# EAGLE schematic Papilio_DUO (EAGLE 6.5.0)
DATABASE: C:/Dropbox/GadgetFactory/GadgetFactory_Engineering/Libraries/GadgetFactory-PARTSDB.txt
Assembly variants: 512KB-SRAM, 1MB-SRAM, 2MB-SRAM, No-SRAM

## Sheet 1 of 4: FPGA
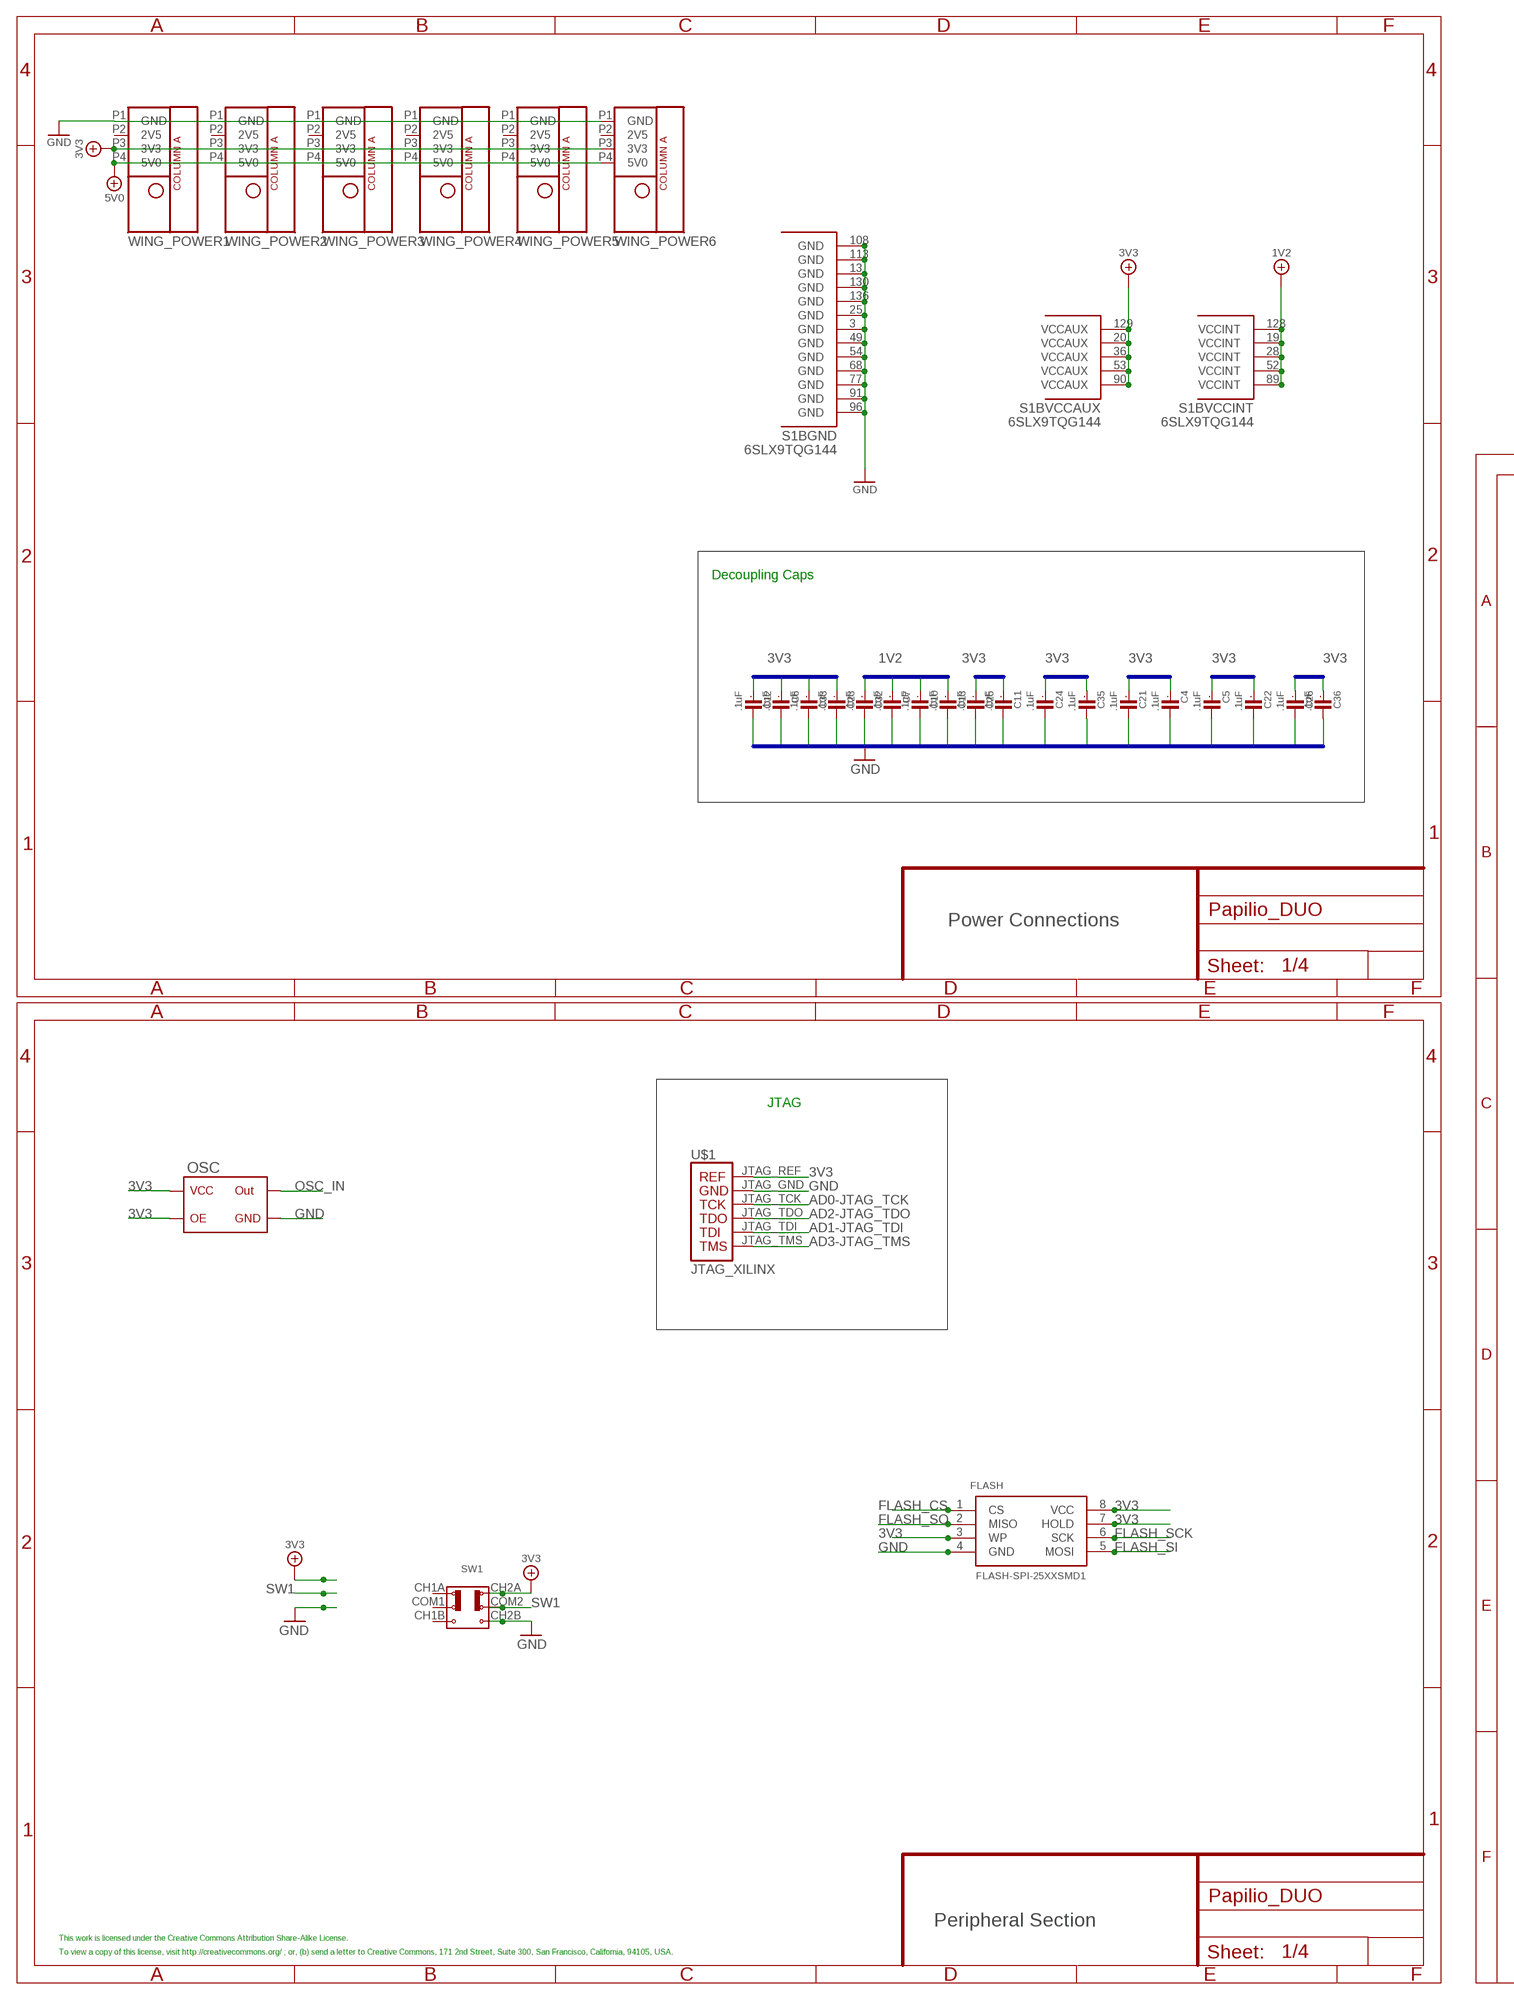
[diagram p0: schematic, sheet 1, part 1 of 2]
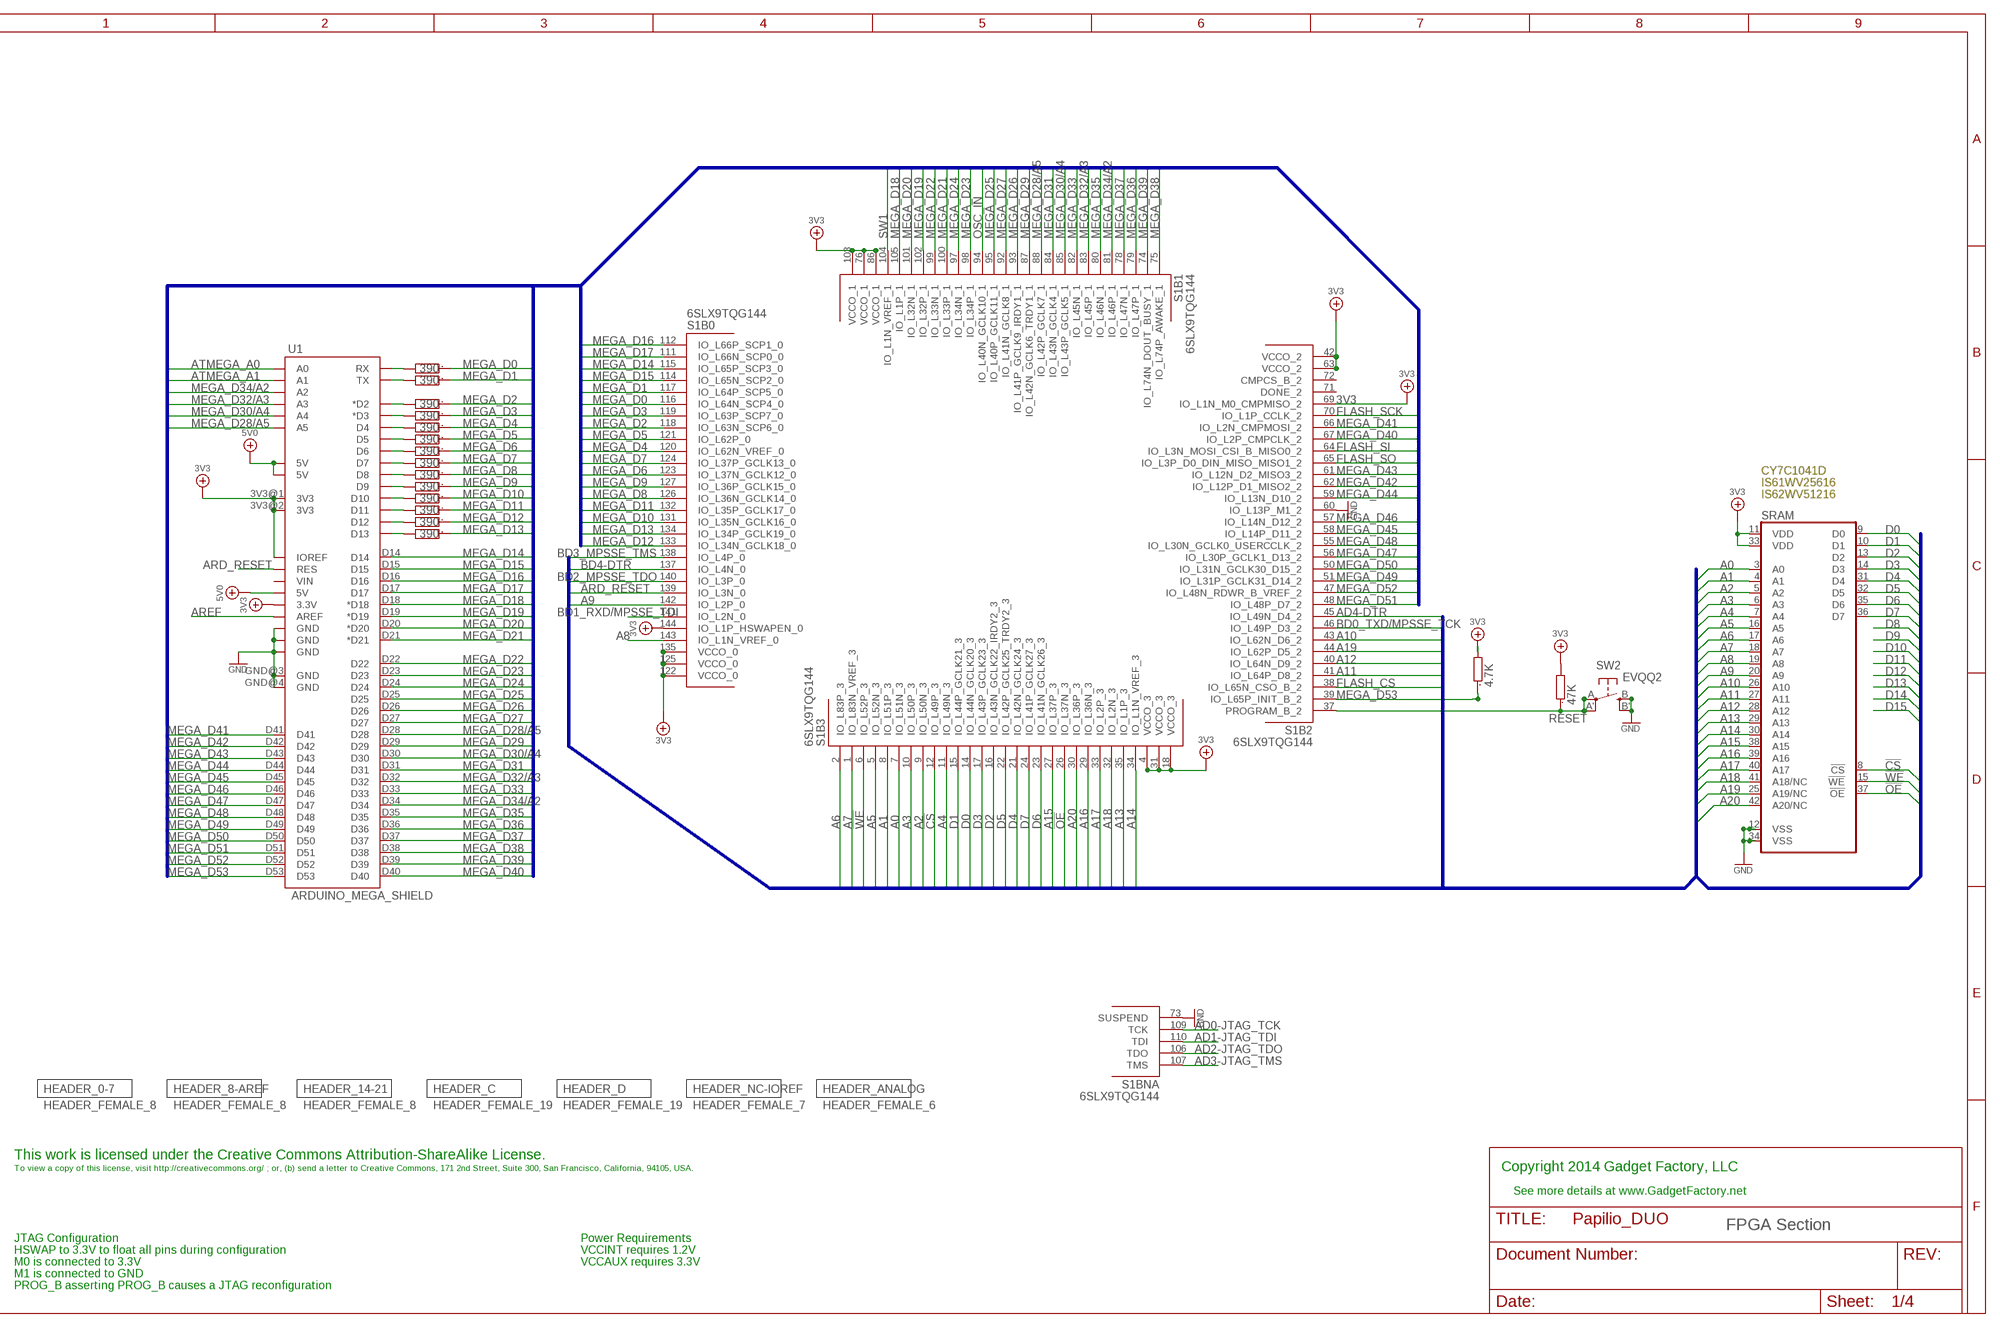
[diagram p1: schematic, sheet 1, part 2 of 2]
HEADER_0-7 (BOM-PART): BOM: INCLUDE; PARTNO: PPTC081LFBN-RC; QTY: 1
HEADER_8-AREF (BOM-PART): BOM: INCLUDE; PARTNO: PPTC081LFBN-RC; QTY: 1
HEADER_14-21 (BOM-PART): BOM: INCLUDE; PARTNO: PPTC081LFBN-RC; QTY: 1
HEADER_ANALOG (BOM-PART): BOM: INCLUDE; PARTNO: PPTC061LFBN-RC; QTY: 1
HEADER_C (BOM-PART): BOM: INCLUDE; PARTNO: PPTC191LFBN-RC; QTY: 1
HEADER_D (BOM-PART): BOM: INCLUDE; PARTNO: PPTC191LFBN-RC; QTY: 1
HEADER_NC-IOREF (BOM-PART): BOM: INCLUDE; PARTNO: PPTC071LFBN-RC; QTY: 1

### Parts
C4  .1uF  C0603  [0603]
C5  .1uF  C0603  [0603]
C6  .1uF  C0603  [0603]
C7  .1uF  C0603  [0603]
C10  .1uF  C0603  [0603]
C11  .1uF  C0603  [0603]
C12  .1uF  C0603  [0603]
C13  .1uF  C0603  [0603]
C21  .1uF  C0603  [0603]
C22  .1uF  C0603  [0603]
C23  .1uF  C0603  [0603]
C24  .1uF  C0603  [0603]
C25  .1uF  C0603  [0603]
C26  .1uF  C0603  [0603]
C32  .1uF  C0603  [0603]
C33  .1uF  C0603  [0603]
C35  .1uF  C0603  [0603]
C36  .1uF  C0603  [0603]
FLASH  FLASH-SPI-25XXSMD1  [SO08-EIAJ]
OSC  OSC1  [OSC1]
R8  390  R0603  [0603]
R9  390  R0603  [0603]
R10  390  R0603  [0603]
R11  390  R0603  [0603]
R12  390  R0603  [0603]
R13  390  R0603  [0603]
R14  390  R0603  [0603]
R15  390  R0603  [0603]
R16  390  R0603  [0603]
R17  390  R0603  [0603]
R18  390  R0603  [0603]
R19  390  R0603  [0603]
R20  390  R0603  [0603]
R21  390  R0603  [0603]
R31  47K  R0805  [0805]
R32  4.7K  R0603  [0603]
S1  6SLX9TQG144  [TQ144]
SRAM  ISSI_SRAM_8BIT  [TSOP44-II]  (variant 512KB-SRAM: 512KB-SRAM)  (variant 1MB-SRAM: 1MB-SRAM)  (variant 2MB-SRAM: 2MB-SRAM)  (not fitted in variant No-SRAM)
SW1  SWITCH-2CH-6P-3010010P1  [6P-2CH-2.54-9.1X3.5X3.2+2H]
SW2  EVQQ2  [EVQ-Q2]
U1  ARDUINO_MEGA_SHIELD  [ARDUINO_MEGA_SHIELD]
U$1  JTAG_XILINX  [JTAG]
WING_POWER1  HEADER_FEMALE_4  POWER_ONLYNOTEXT  [POWER_NO_TEXT]
WING_POWER2  HEADER_FEMALE_4  POWER_ONLYNOTEXT  [POWER_NO_TEXT]
WING_POWER3  HEADER_FEMALE_4  POWER_ONLYNOTEXT  [POWER_NO_TEXT]
WING_POWER4  HEADER_FEMALE_4  POWER_ONLYNOTEXT  [POWER_NO_TEXT]
WING_POWER5  HEADER_FEMALE_4  POWER_ONLYNOTEXT  [POWER_NO_TEXT]
WING_POWER6  HEADER_FEMALE_4  POWER_ONLYNOTEXT  [POWER_NO_TEXT]

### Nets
1V2: C7.1 C10.1 C13.1 C32.1 S1.19(BVCCINT:VCCINT) S1.28(BVCCINT:VCCINT) S1.52(BVCCINT:VCCINT) S1.89(BVCCINT:VCCINT) S1.128(BVCCINT:VCCINT) ; also sheet 2
3V3: C4.1 C5.1 C6.1 C11.1 C12.1 C21.1 C22.1 C23.1 C24.1 C25.1 C26.1 C33.1 C35.1 C36.1 FLASH.3(WP) FLASH.7(HOLD) FLASH.8(VCC) OSC.1@1(OE) OSC.4@4(VCC) R31.2 R32.2 S1.4(B3:VCCO_3) S1.18(B3:VCCO_3) S1.20(BVCCAUX:VCCAUX) S1.31(B3:VCCO_3) S1.36(BVCCAUX:VCCAUX) S1.42(B2:VCCO_2) S1.53(BVCCAUX:VCCAUX) S1.63(B2:VCCO_2) S1.69(B2:IO_L1N_M0_CMPMISO_2) S1.76(B1:VCCO_1) S1.86(B1:VCCO_1) S1.90(BVCCAUX:VCCAUX) S1.103(B1:VCCO_1) S1.122(B0:VCCO_0) S1.125(B0:VCCO_0) S1.129(BVCCAUX:VCCAUX) S1.135(B0:VCCO_0) S1.144(B0:IO_L1P_HSWAPEN_0) SRAM.11(VDD) SRAM.33(VDD) SW1.CH2A U1.3.3V U1.3V3@1(3V3) U1.3V3@2(3V3) U1.IOREF U$1.JTAG_REF WING_POWER1.P3(3V3) WING_POWER2.P3(3V3) WING_POWER3.P3(3V3) WING_POWER4.P3(3V3) WING_POWER5.P3(3V3) WING_POWER6.P3(3V3) ; also sheet 2,3,4
5V0: U1.5V@0(5V) U1.5V@1(5V) U1.5V@2(5V) WING_POWER1.P4(5V0) WING_POWER2.P4(5V0) WING_POWER3.P4(5V0) WING_POWER4.P4(5V0) WING_POWER5.P4(5V0) WING_POWER6.P4(5V0) ; also sheet 2
!CS: S1.12(B3:IO_L49P_3) SRAM.8(!CS)
!OE: S1.26(B3:IO_L37N_3) SRAM.37(!OE)
!WE: S1.6(B3:IO_L52P_3) SRAM.15(!WE)
A0: S1.7(B3:IO_L51N_3) SRAM.3(A0)
A1: S1.8(B3:IO_L51P_3) SRAM.4(A1)
A2: S1.9(B3:IO_L50N_3) SRAM.5(A2)
A3: S1.10(B3:IO_L50P_3) SRAM.6(A3)
A4: S1.11(B3:IO_L49N_3) SRAM.7(A4)
A5: S1.5(B3:IO_L52N_3) SRAM.16(A5)
A6: S1.2(B3:IO_L83P_3) SRAM.17(A6)
A7: S1.1(B3:IO_L83N_VREF_3) SRAM.18(A7)
A8: S1.143(B0:IO_L1N_VREF_0) SRAM.19(A8)
A9: S1.142(B0:IO_L2P_0) SRAM.20(A9)
A10: S1.43(B2:IO_L62N_D6_2) SRAM.26(A10)
A11: S1.41(B2:IO_L64P_D8_2) SRAM.27(A11)
A12: S1.40(B2:IO_L64N_D9_2) SRAM.28(A12)
A13: S1.35(B3:IO_L1P_3) SRAM.29(A13)
A14: S1.34(B3:IO_L1N_VREF_3) SRAM.30(A14)
A15: S1.27(B3:IO_L37P_3) SRAM.38(A15)
A16: S1.29(B3:IO_L36N_3) SRAM.39(A16)
A17: S1.33(B3:IO_L2P_3) SRAM.40(A17)
A18: S1.32(B3:IO_L2N_3) SRAM.41(A18/NC)
A19: S1.44(B2:IO_L62P_D5_2) SRAM.25(A19/NC)
A20: S1.30(B3:IO_L36P_3) SRAM.42(A20/NC)
AD0-JTAG_TCK: S1.109(BNA:TCK) U$1.JTAG_TCK ; also sheet 3
AD1-JTAG_TDI: S1.110(BNA:TDI) U$1.JTAG_TDI ; also sheet 3
AD2-JTAG_TDO: S1.106(BNA:TDO) U$1.JTAG_TDO ; also sheet 3
AD3-JTAG_TMS: S1.107(BNA:TMS) U$1.JTAG_TMS ; also sheet 3
AD4-DTR: S1.45(B2:IO_L49N_D4_2) ; also sheet 3
ARD_RESET: S1.139(B0:IO_L3N_0) U1.RES ; also sheet 4
AREF [aref]: U1.AREF ; also sheet 4
ATMEGA_A0: U1.A0 ; also sheet 4
ATMEGA_A1: U1.A1 ; also sheet 4
ATMEGA_D0/RX: R21.2 U1.RX ; also sheet 4
ATMEGA_D1/TX: R20.2 U1.TX ; also sheet 4
ATMEGA_D2: R19.2 U1.D2(*D2) ; also sheet 4
ATMEGA_D3: R18.2 U1.D3(*D3) ; also sheet 4
ATMEGA_D4: R17.2 U1.D4 ; also sheet 4
ATMEGA_D5*: R16.2 U1.D5 ; also sheet 4
ATMEGA_D6*: R15.2 U1.D6 ; also sheet 4
ATMEGA_D7: R14.2 U1.D7 ; also sheet 4
ATMEGA_IO8: R13.2 U1.D8 ; also sheet 4
ATMEGA_IO9*: R12.2 U1.D9 ; also sheet 4
ATMEGA_IO10*: R11.2 U1.D10 ; also sheet 4
ATMEGA_IO11*: R10.2 U1.D11 ; also sheet 4
ATMEGA_IO12: R9.2 U1.D12 ; also sheet 4
ATMEGA_IO13*: R8.2 U1.D13 ; also sheet 4
BD0_TXD/MPSSE_TCK: S1.46(B2:IO_L49P_D3_2) ; also sheet 3
BD1_RXD/MPSSE_TDI: S1.141(B0:IO_L2N_0) ; also sheet 3
BD2_MPSSE_TDO: S1.140(B0:IO_L3P_0) ; also sheet 3
BD3_MPSSE_TMS: S1.138(B0:IO_L4P_0) ; also sheet 3
BD4-DTR: S1.137(B0:IO_L4N_0) ; also sheet 3
D0: S1.14(B3:IO_L44N_GCLK20_3) SRAM.9(D0)
D1: S1.15(B3:IO_L44P_GCLK21_3) SRAM.10(D1)
D2: S1.16(B3:IO_L43N_GCLK22_IRDY2_3) SRAM.13(D2)
D3: S1.17(B3:IO_L43P_GCLK23_3) SRAM.14(D3)
D4: S1.21(B3:IO_L42N_GCLK24_3) SRAM.31(D4)
D5: S1.22(B3:IO_L42P_GCLK25_TRDY2_3) SRAM.32(D5)
D6: S1.23(B3:IO_L41N_GCLK26_3) SRAM.35(D6)
D7: S1.24(B3:IO_L41P_GCLK27_3) SRAM.36(D7)
FLASH_CS: FLASH.1(CS) S1.38(B2:IO_L65N_CSO_B_2)
FLASH_SCK: FLASH.6(SCK) S1.70(B2:IO_L1P_CCLK_2)
FLASH_SI: FLASH.5(MOSI) S1.64(B2:IO_L3N_MOSI_CSI_B_MISO0_2)
FLASH_SO: FLASH.2(MISO) S1.65(B2:IO_L3P_D0_DIN_MISO_MISO1_2)
GND: C4.2 C5.2 C6.2 C7.2 C10.2 C11.2 C12.2 C13.2 C21.2 C22.2 C23.2 C24.2 C25.2 C26.2 C32.2 C33.2 C35.2 C36.2 FLASH.4(GND) OSC.2@2(GND) S1.3(BGND:GND) S1.13(BGND:GND) S1.25(BGND:GND) S1.49(BGND:GND) S1.54(BGND:GND) S1.60(B2:IO_L13P_M1_2) S1.68(BGND:GND) S1.73(BNA:SUSPEND) S1.77(BGND:GND) S1.91(BGND:GND) S1.96(BGND:GND) S1.108(BGND:GND) S1.113(BGND:GND) S1.130(BGND:GND) S1.136(BGND:GND) SRAM.12(VSS) SRAM.34(VSS) SW1.CH2B SW2.B'(S1) SW2.B(S) U1.GND@0(GND) U1.GND@1(GND) U1.GND@2(GND) U1.GND@3(GND) U1.GND@4(GND) U$1.JTAG_GND WING_POWER1.P1(GND) WING_POWER2.P1(GND) WING_POWER3.P1(GND) WING_POWER4.P1(GND) WING_POWER5.P1(GND) WING_POWER6.P1(GND) ; also sheet 2,3,4
MEGA_D0: R21.1 S1.116(B0:IO_L64N_SCP4_0)
MEGA_D1: R20.1 S1.117(B0:IO_L64P_SCP5_0)
MEGA_D2: R19.1 S1.118(B0:IO_L63N_SCP6_0)
MEGA_D3: R18.1 S1.119(B0:IO_L63P_SCP7_0)
MEGA_D4: R17.1 S1.120(B0:IO_L62N_VREF_0)
MEGA_D5: R16.1 S1.121(B0:IO_L62P_0)
MEGA_D6: R15.1 S1.123(B0:IO_L37N_GCLK12_0)
MEGA_D7: R14.1 S1.124(B0:IO_L37P_GCLK13_0)
MEGA_D8: R13.1 S1.126(B0:IO_L36N_GCLK14_0)
MEGA_D9: R12.1 S1.127(B0:IO_L36P_GCLK15_0)
MEGA_D10: R11.1 S1.131(B0:IO_L35N_GCLK16_0)
MEGA_D11: R10.1 S1.132(B0:IO_L35P_GCLK17_0)
MEGA_D12: R9.1 S1.133(B0:IO_L34N_GCLK18_0)
MEGA_D13: R8.1 S1.134(B0:IO_L34P_GCLK19_0)
MEGA_D14: S1.115(B0:IO_L65P_SCP3_0) U1.D14 ; also sheet 4
MEGA_D15: S1.114(B0:IO_L65N_SCP2_0) U1.D15 ; also sheet 4
MEGA_D16: S1.112(B0:IO_L66P_SCP1_0) U1.D16 ; also sheet 4
MEGA_D17: S1.111(B0:IO_L66N_SCP0_0) U1.D17
MEGA_D18: S1.105(B1:IO_L1P_1) U1.D18(*D18)
MEGA_D19: S1.102(B1:IO_L32P_1) U1.D19(*D19)
MEGA_D20: S1.101(B1:IO_L32N_1) U1.D20(*D20)
MEGA_D21: S1.100(B1:IO_L33P_1) U1.D21(*D21)
MEGA_D22: S1.99(B1:IO_L33N_1) U1.D22
MEGA_D23: S1.98(B1:IO_L34P_1) U1.D23
MEGA_D24: S1.97(B1:IO_L34N_1) U1.D24
MEGA_D25: S1.95(B1:IO_L40P_GCLK11_1) U1.D25
MEGA_D26: S1.93(B1:IO_L41P_GCLK9_IRDY1_1) U1.D26
MEGA_D27: S1.92(B1:IO_L41N_GCLK8_1) U1.D27
MEGA_D28/A5: S1.88(B1:IO_L42P_GCLK7_1) U1.A5 U1.D28 ; also sheet 4
MEGA_D29: S1.87(B1:IO_L42N_GCLK6_TRDY1_1) U1.D29
MEGA_D30/A4: S1.85(B1:IO_L43P_GCLK5_1) U1.A4 U1.D30 ; also sheet 4
MEGA_D31: S1.84(B1:IO_L43N_GCLK4_1) U1.D31
MEGA_D32/A3: S1.83(B1:IO_L45P_1) U1.A3 U1.D32 ; also sheet 4
MEGA_D33: S1.82(B1:IO_L45N_1) U1.D33
MEGA_D34/A2: S1.81(B1:IO_L46P_1) U1.A2 U1.D34 ; also sheet 4
MEGA_D35: S1.80(B1:IO_L46N_1) U1.D35
MEGA_D36: S1.79(B1:IO_L47P_1) U1.D36
MEGA_D37: S1.78(B1:IO_L47N_1) U1.D37
MEGA_D38: S1.75(B1:IO_L74P_AWAKE_1) U1.D38
MEGA_D39: S1.74(B1:IO_L74N_DOUT_BUSY_1) U1.D39
MEGA_D40: S1.67(B2:IO_L2P_CMPCLK_2) U1.D40
MEGA_D41: S1.66(B2:IO_L2N_CMPMOSI_2) U1.D41
MEGA_D42: S1.62(B2:IO_L12P_D1_MISO2_2) U1.D42
MEGA_D43: S1.61(B2:IO_L12N_D2_MISO3_2) U1.D43
MEGA_D44: S1.59(B2:IO_L13N_D10_2) U1.D44
MEGA_D45: S1.58(B2:IO_L14P_D11_2) U1.D45
MEGA_D46: S1.57(B2:IO_L14N_D12_2) U1.D46
MEGA_D47: S1.56(B2:IO_L30P_GCLK1_D13_2) U1.D47
MEGA_D48: S1.55(B2:IO_L30N_GCLK0_USERCCLK_2) U1.D48
MEGA_D49: S1.51(B2:IO_L31P_GCLK31_D14_2) U1.D49
MEGA_D50: S1.50(B2:IO_L31N_GCLK30_D15_2) U1.D50
MEGA_D51: S1.48(B2:IO_L48P_D7_2) U1.D51
MEGA_D52: S1.47(B2:IO_L48N_RDWR_B_VREF_2) U1.D52
MEGA_D53: R32.1 S1.39(B2:IO_L65P_INIT_B_2) U1.D53
OSC_IN: OSC.3@3(OUT) S1.94(B1:IO_L40N_GCLK10_1)
RESET: R31.1 S1.37(B2:PROGRAM_B_2) SW2.A'(P1) SW2.A(P)
SW1: S1.104(B1:IO_L1N_VREF_1) SW1.COM2
Unconnected: S1.71(B2:DONE_2) S1.72(B2:CMPCS_B_2) SW1.CH1A SW1.CH1B SW1.COM1 U1.VIN WING_POWER1.P2(2V5) WING_POWER2.P2(2V5) WING_POWER3.P2(2V5) WING_POWER4.P2(2V5) WING_POWER5.P2(2V5) WING_POWER6.P2(2V5)

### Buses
GND
1V2
MEGA_A[0..15],MEGA_D[0..53],W1_B[1..16],OSC_IN,FLASH_SCK,FLASH_SI,FLASH_SO,FLASH_CS,USB_TXD,USB_RXD,LED1,LED2,LED3,LED4
3V3
A[0..20],D[0..15],CS,WE,OE,BE,LED4

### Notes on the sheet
- Decoupling Caps
- Power Connections
- CY7C1041D
- IS61WV25616
- IS62WV51216
- JTAG
- RESET
- This work is licensed under the Creative Commons Attribution-ShareAlike License.
- To view a copy of this license, visit http://creativecommons.org/ ; or, (b) send a letter to Creative Commons, 171 2nd Street, Suite 300, San Francisco, California, 94105, USA. | Copyright 2014 Gadget Factory, LLC
- See more details at www.GadgetFactory.net
- FPGA Section
- JTAG Configuration | Power Requirements
- HSWAP to 3.3V to float all pins during configuration | VCCINT requires 1.2V
- Peripheral Section | M0 is connected to 3.3V | VCCAUX requires 3.3V
- This work is licensed under the Creative Commons Attribution Share-Alike License. | M1 is connected to GND
- To view a copy of this license, visit http://creativecommons.org/ ; or, (b) send a letter to Creative Commons, 171 2nd Street, Suite 300, San Francisco, California, 94105, USA. | PROG_B asserting PROG_B causes a JTAG reconfiguration

## Sheet 2 of 4: Power
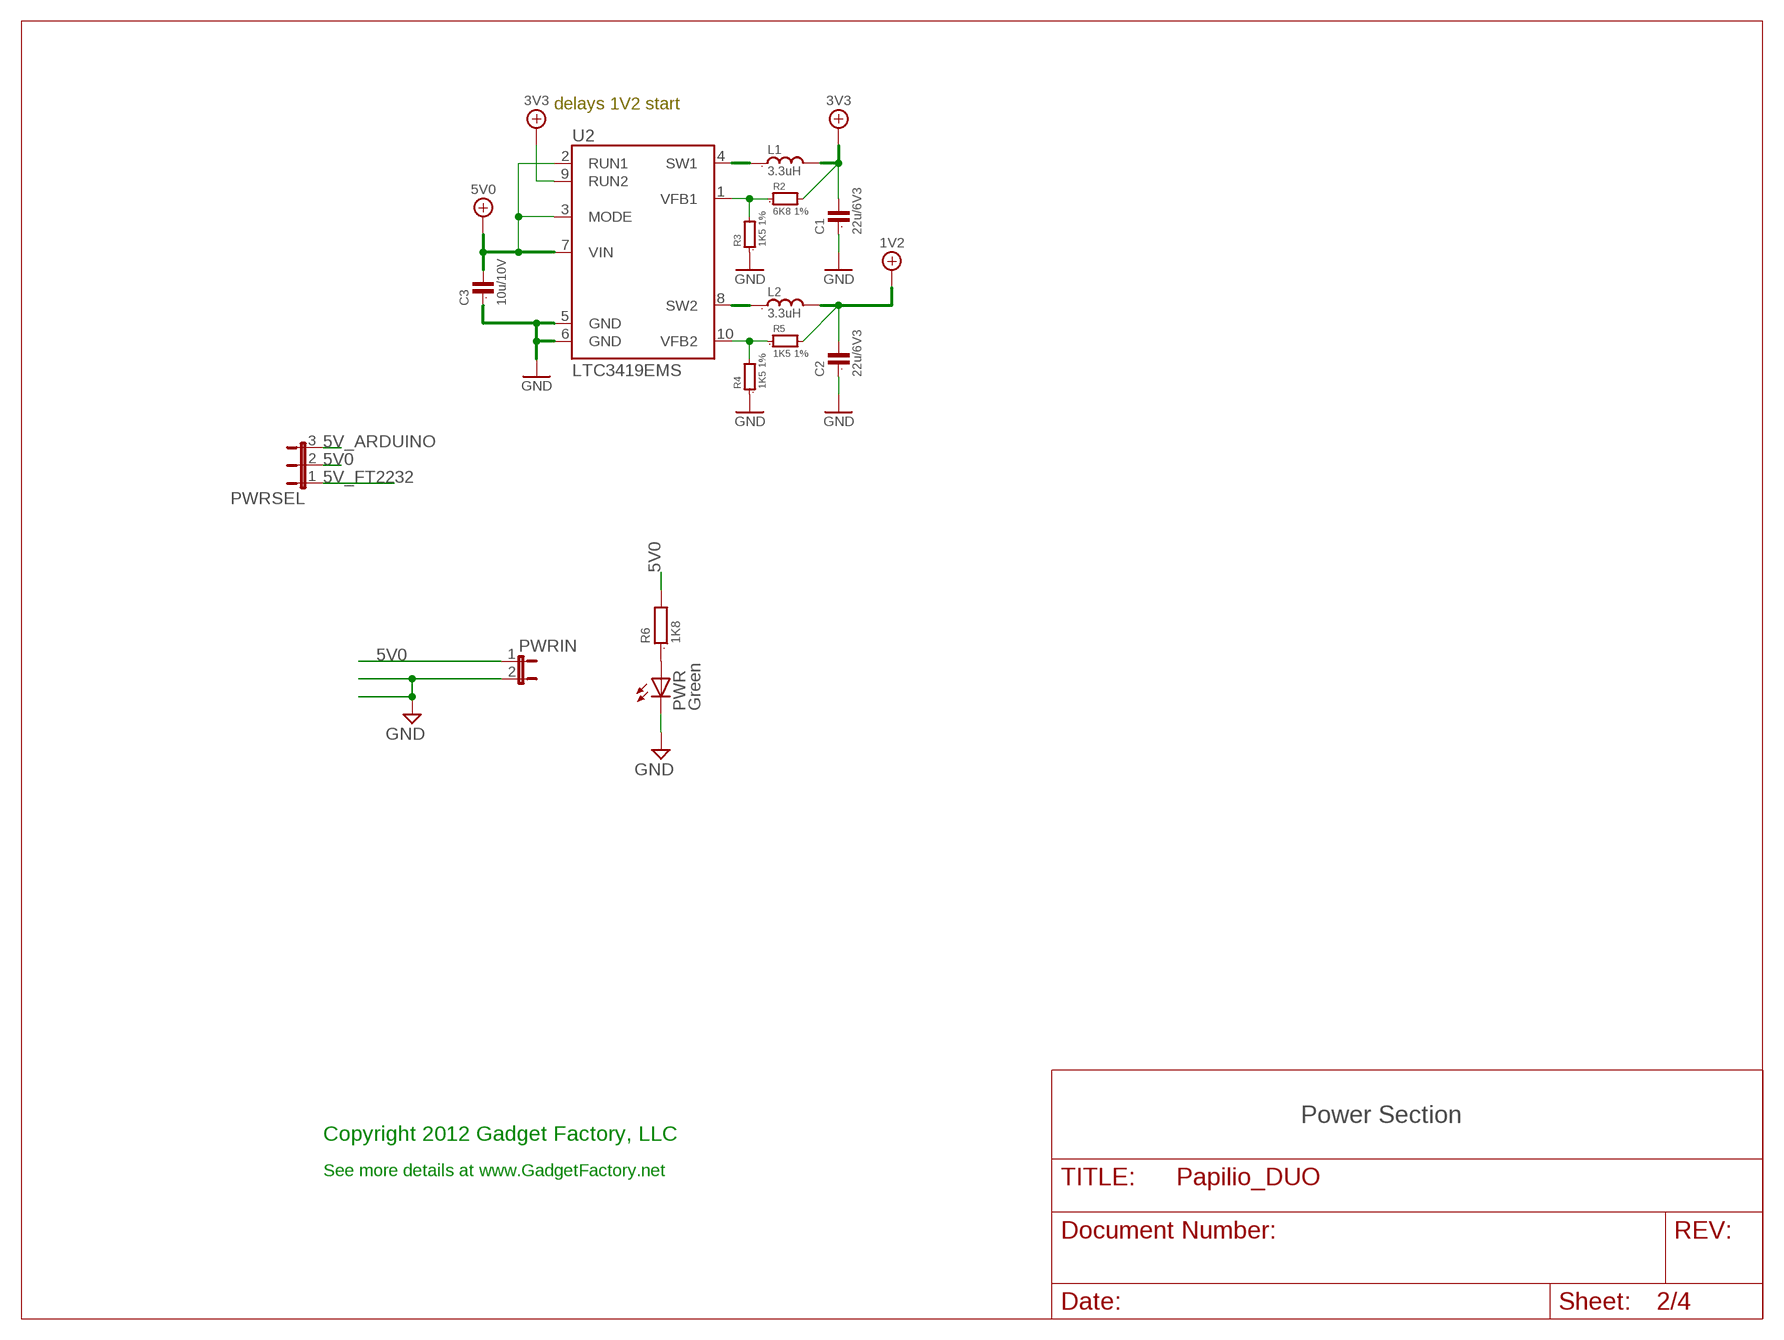
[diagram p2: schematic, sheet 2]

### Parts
C1  22u/6V3  C0805  [0805]
C2  22u/6V3  C0805  [0805]
C3  10u/10V  C0805  [0805]
L1  3.3uH  L_VLS3015  [VLS3015]
L2  3.3uH  L_VLS3015  [VLS3015]
PWR  Green  LEDCHIP-LED0805  [CHIP-LED0805]
PWRIN  JP1E  [JP1]
PWRSEL  JP2E  [JP2]
R2  6K8 1%  R-SMALL0603  [0603]
R3  1K5 1%  R-SMALL0603  [0603]
R4  1K5 1%  R-SMALL0603  [0603]
R5  1K5 1%  R-SMALL0603  [0603]
R6  1K8  R0603  [0603]
U2  LTC3419EMS  [MSOP10]

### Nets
1V2: C2.2 L2.2 R5.2 ; also sheet 1
3V3: C1.2 L1.2 R2.2 U2.9(RUN2) ; also sheet 1,3,4
5V0: C3.2 PWRIN.1 PWRSEL.2 R6.2 U2.2(RUN1) U2.3(MODE) U2.7(VIN) ; also sheet 1
5V_ARDUINO: PWRSEL.3 ; also sheet 4
5V_FT2232: PWRSEL.1 ; also sheet 3
FB_1V2: R4.2 R5.1 U2.10(VFB2)
FB_3V3: R2.1 R3.2 U2.1(VFB1)
GND: C1.1 C2.1 C3.1 PWR.C PWRIN.2 R3.1 R4.1 U2.5(GND) U2.6(GND) ; also sheet 1,3,4
N$8: PWR.A R6.1
SW_1V2: L2.1 U2.8(SW2)
SW_3V3: L1.1 U2.4(SW1)

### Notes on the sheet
- delays 1V2 start
- Power Section
- Copyright 2012 Gadget Factory, LLC
- See more details at www.GadgetFactory.net

## Sheet 3 of 4: FT2232H
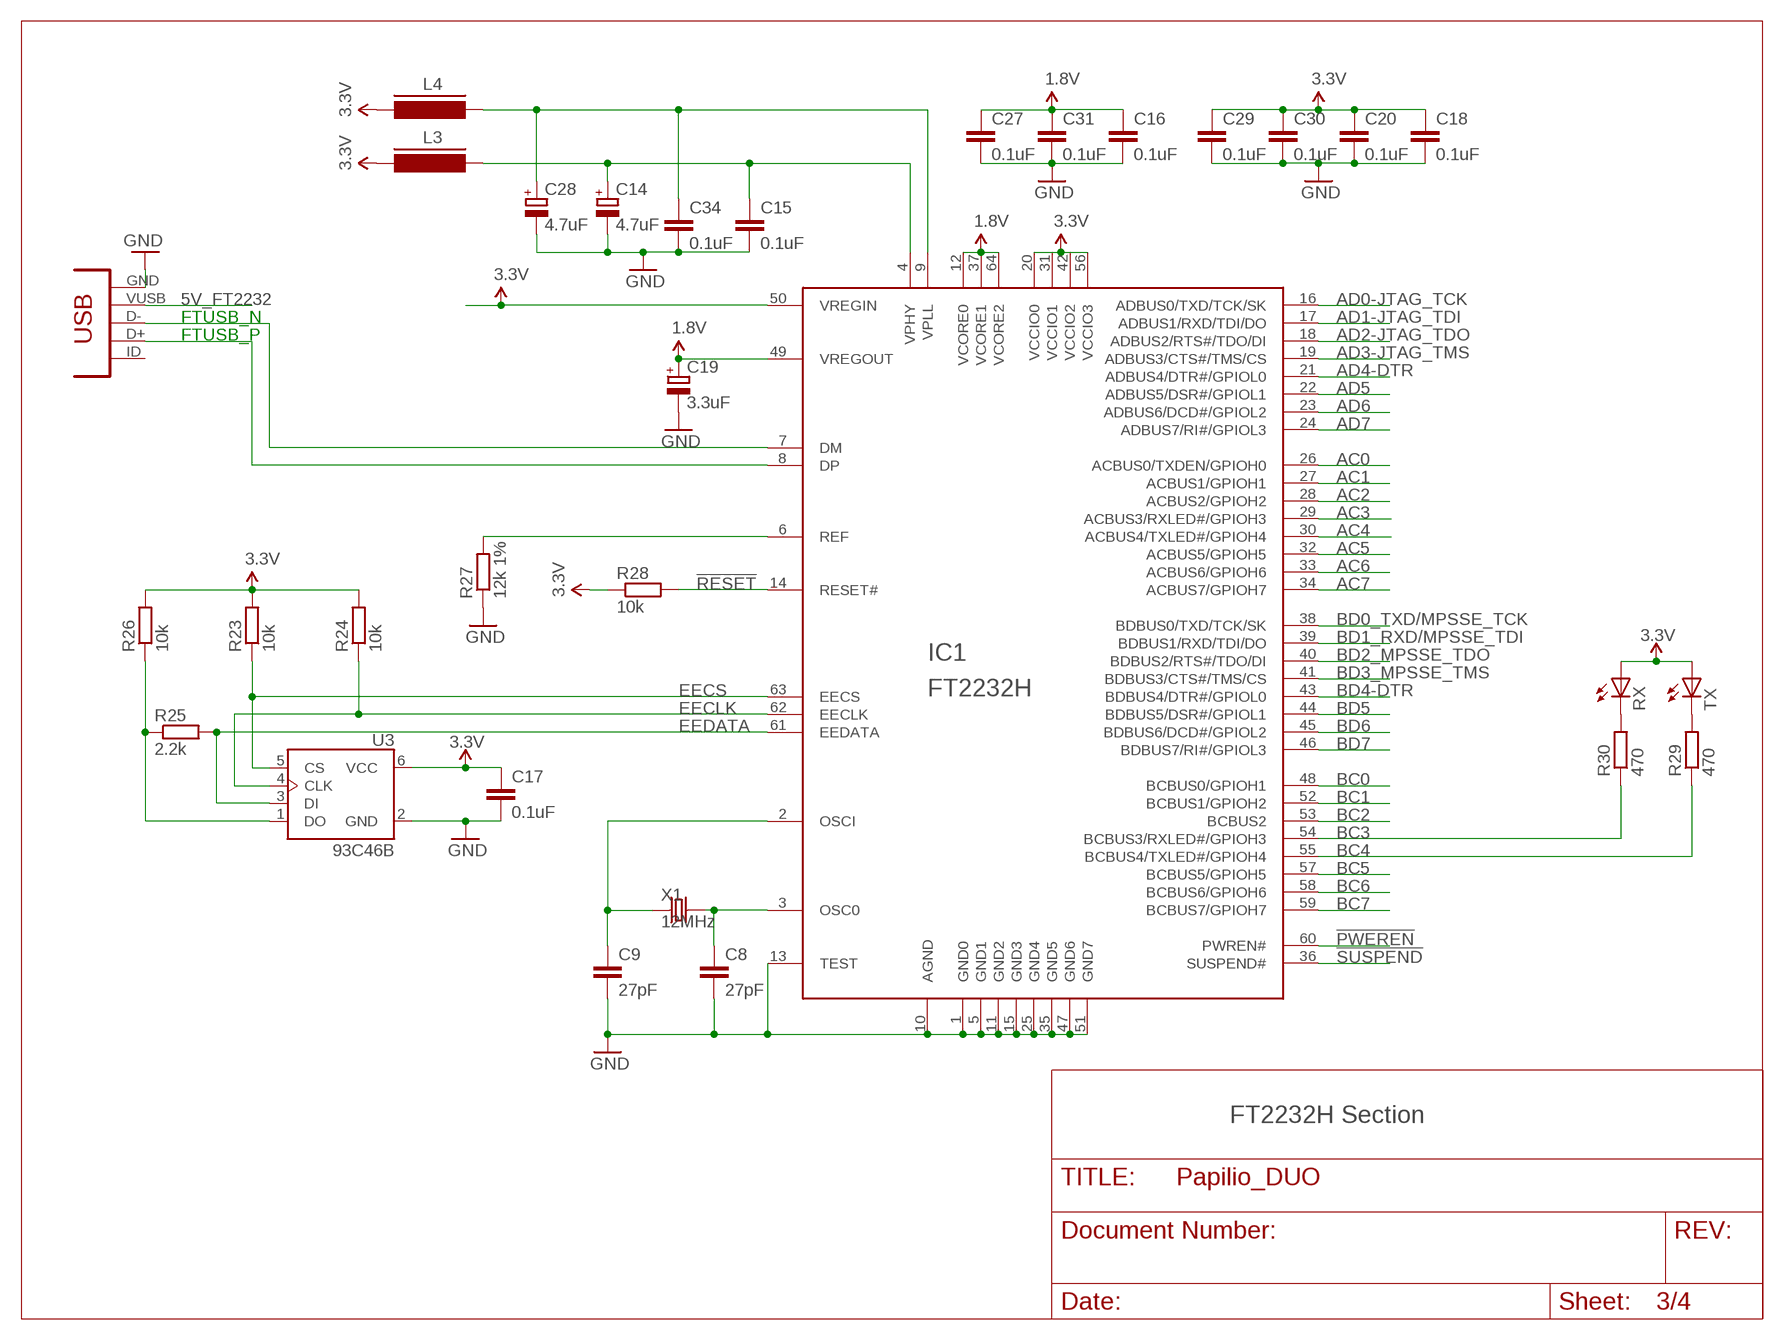
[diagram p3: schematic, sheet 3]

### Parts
C8  27pF  CAPC603  [C603]
C9  27pF  CAPC603  [C603]
C14  4.7uF  CAP_POLSMC_A  [SMC_A]
C15  0.1uF  CAPC603  [C603]
C16  0.1uF  CAPC603  [C603]
C17  0.1uF  CAPC603  [C603]
C18  0.1uF  CAPC603  [C603]
C19  3.3uF  CAP_POLSMC_A  [SMC_A]
C20  0.1uF  CAPC603  [C603]
C27  0.1uF  CAPC603  [C603]
C28  4.7uF  CAP_POLSMC_A  [SMC_A]
C29  0.1uF  CAPC603  [C603]
C30  0.1uF  CAPC603  [C603]
C31  0.1uF  CAPC603  [C603]
C34  0.1uF  CAPC603  [C603]
FPGAUSB  CONN_USB  [CONN_USB_MINI-B]
IC1  FT2232H  [LQFP64]
L3  FERRITE_BEAD603  [FB603]
L4  FERRITE_BEAD603  [FB603]
R23  10k  RESISTORR603  [R603]
R24  10k  RESISTORR603  [R603]
R25  2.2k  RESISTORR603  [R603]
R26  10k  RESISTORR603  [R603]
R27  12k 1%  RESISTORR603  [R603]
R28  10k  RESISTORR603  [R603]
R29  470  RESISTORR603  [R603]
R30  470  RESISTORR603  [R603]
RX  LED805  [LED-805]
TX  LED805  [LED-805]
U3  93C46B  DIGITAL-EEPROM-MICROWIRE-6P_SOT23  [SOT23-6]
X1  12MHz  CRYSTAL_212M_  [4X6]

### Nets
1.8V: C16.1 C19.+ C27.1 C31.1 IC1.12(VCORE0) IC1.37(VCORE1) IC1.49(VREGOUT) IC1.64(VCORE2)
3V3: C17.1 C18.1 C20.1 C29.1 C30.1 IC1.20(VCCIO0) IC1.31(VCCIO1) IC1.42(VCCIO2) IC1.50(VREGIN) IC1.56(VCCIO3) L3.2 L4.2 R23.2 R24.2 R26.2 R28.1 RX.A TX.A U3.6(VCC) ; supply symbol labelled 3.3V ; also sheet 1,2,4
5V_FT2232: FPGAUSB.VUSB ; also sheet 2
!PWEREN: IC1.60(PWREN#)
!RESET: IC1.14(RESET#) R28.2
!SUSPEND: IC1.36(SUSPEND#)
AC0: IC1.26(ACBUS0/TXDEN/GPIOH0)
AC1: IC1.27(ACBUS1/GPIOH1)
AC2: IC1.28(ACBUS2/GPIOH2)
AC3: IC1.29(ACBUS3/RXLED#/GPIOH3)
AC4: IC1.30(ACBUS4/TXLED#/GPIOH4)
AC5: IC1.32(ACBUS5/GPIOH5)
AC6: IC1.33(ACBUS6/GPIOH6)
AC7: IC1.34(ACBUS7/GPIOH7)
AD0-JTAG_TCK: IC1.16(ADBUS0/TXD/TCK/SK) ; also sheet 1
AD1-JTAG_TDI: IC1.17(ADBUS1/RXD/TDI/DO) ; also sheet 1
AD2-JTAG_TDO: IC1.18(ADBUS2/RTS#/TDO/DI) ; also sheet 1
AD3-JTAG_TMS: IC1.19(ADBUS3/CTS#/TMS/CS) ; also sheet 1
AD4-DTR: IC1.21(ADBUS4/DTR#/GPIOL0) ; also sheet 1
AD5: IC1.22(ADBUS5/DSR#/GPIOL1)
AD6: IC1.23(ADBUS6/DCD#/GPIOL2)
AD7: IC1.24(ADBUS7/RI#/GPIOL3)
BC0: IC1.48(BCBUS0/GPIOH1)
BC1: IC1.52(BCBUS1/GPIOH2)
BC2: IC1.53(BCBUS2)
BC3: IC1.54(BCBUS3/RXLED#/GPIOH3) R30.1
BC4: IC1.55(BCBUS4/TXLED#/GPIOH4) R29.1
BC5: IC1.57(BCBUS5/GPIOH5)
BC6: IC1.58(BCBUS6/GPIOH6)
BC7: IC1.59(BCBUS7/GPIOH7)
BD0_TXD/MPSSE_TCK: IC1.38(BDBUS0/TXD/TCK/SK) ; also sheet 1
BD1_RXD/MPSSE_TDI: IC1.39(BDBUS1/RXD/TDI/DO) ; also sheet 1
BD2_MPSSE_TDO: IC1.40(BDBUS2/RTS#/TDO/DI) ; also sheet 1
BD3_MPSSE_TMS: IC1.41(BDBUS3/CTS#/TMS/CS) ; also sheet 1
BD4-DTR: IC1.43(BDBUS4/DTR#/GPIOL0) ; also sheet 1
BD5: IC1.44(BDBUS5/DSR#/GPIOL1)
BD6: IC1.45(BDBUS6/DCD#/GPIOL2)
BD7: IC1.46(BDBUS7/RI#/GPIOL3)
EECLK: IC1.62(EECLK) R24.1 U3.4(CLK)
EECS: IC1.63(EECS) R23.1 U3.5(CS)
EEDATA: IC1.61(EEDATA) R25.2 U3.3(DI)
FTUSB_N: FPGAUSB.D- IC1.7(DM)
FTUSB_P: FPGAUSB.D+ IC1.8(DP)
GND: C8.2 C9.2 C14.- C15.2 C16.2 C17.2 C18.2 C19.- C20.2 C27.2 C28.- C29.2 C30.2 C31.2 C34.2 FPGAUSB.GND IC1.1(GND0) IC1.5(GND1) IC1.10(AGND) IC1.11(GND2) IC1.13(TEST) IC1.15(GND3) IC1.25(GND4) IC1.35(GND5) IC1.47(GND6) IC1.51(GND7) R27.1 U3.2(GND) ; also sheet 1,2,4
N$9: IC1.6(REF) R27.2
N$22: C9.1 IC1.2(OSCI) X1.1(X1)
N$23: C8.1 IC1.3(OSC0) X1.2(X2)
N$24: R30.2 RX.C
N$25: R29.2 TX.C
N$45: R25.1 R26.1 U3.1(DO)
N$48: C14.+ C15.1 IC1.4(VPHY) L3.1
N$49: C28.+ C34.1 IC1.9(VPLL) L4.1
Unconnected: FPGAUSB.BODY@1(BODY) FPGAUSB.BODY@2(BODY) FPGAUSB.BODY@3(BODY) FPGAUSB.BODY@4(BODY) FPGAUSB.ID(USBID)

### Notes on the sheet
- FT2232H Section

## Sheet 4 of 4: Arduino
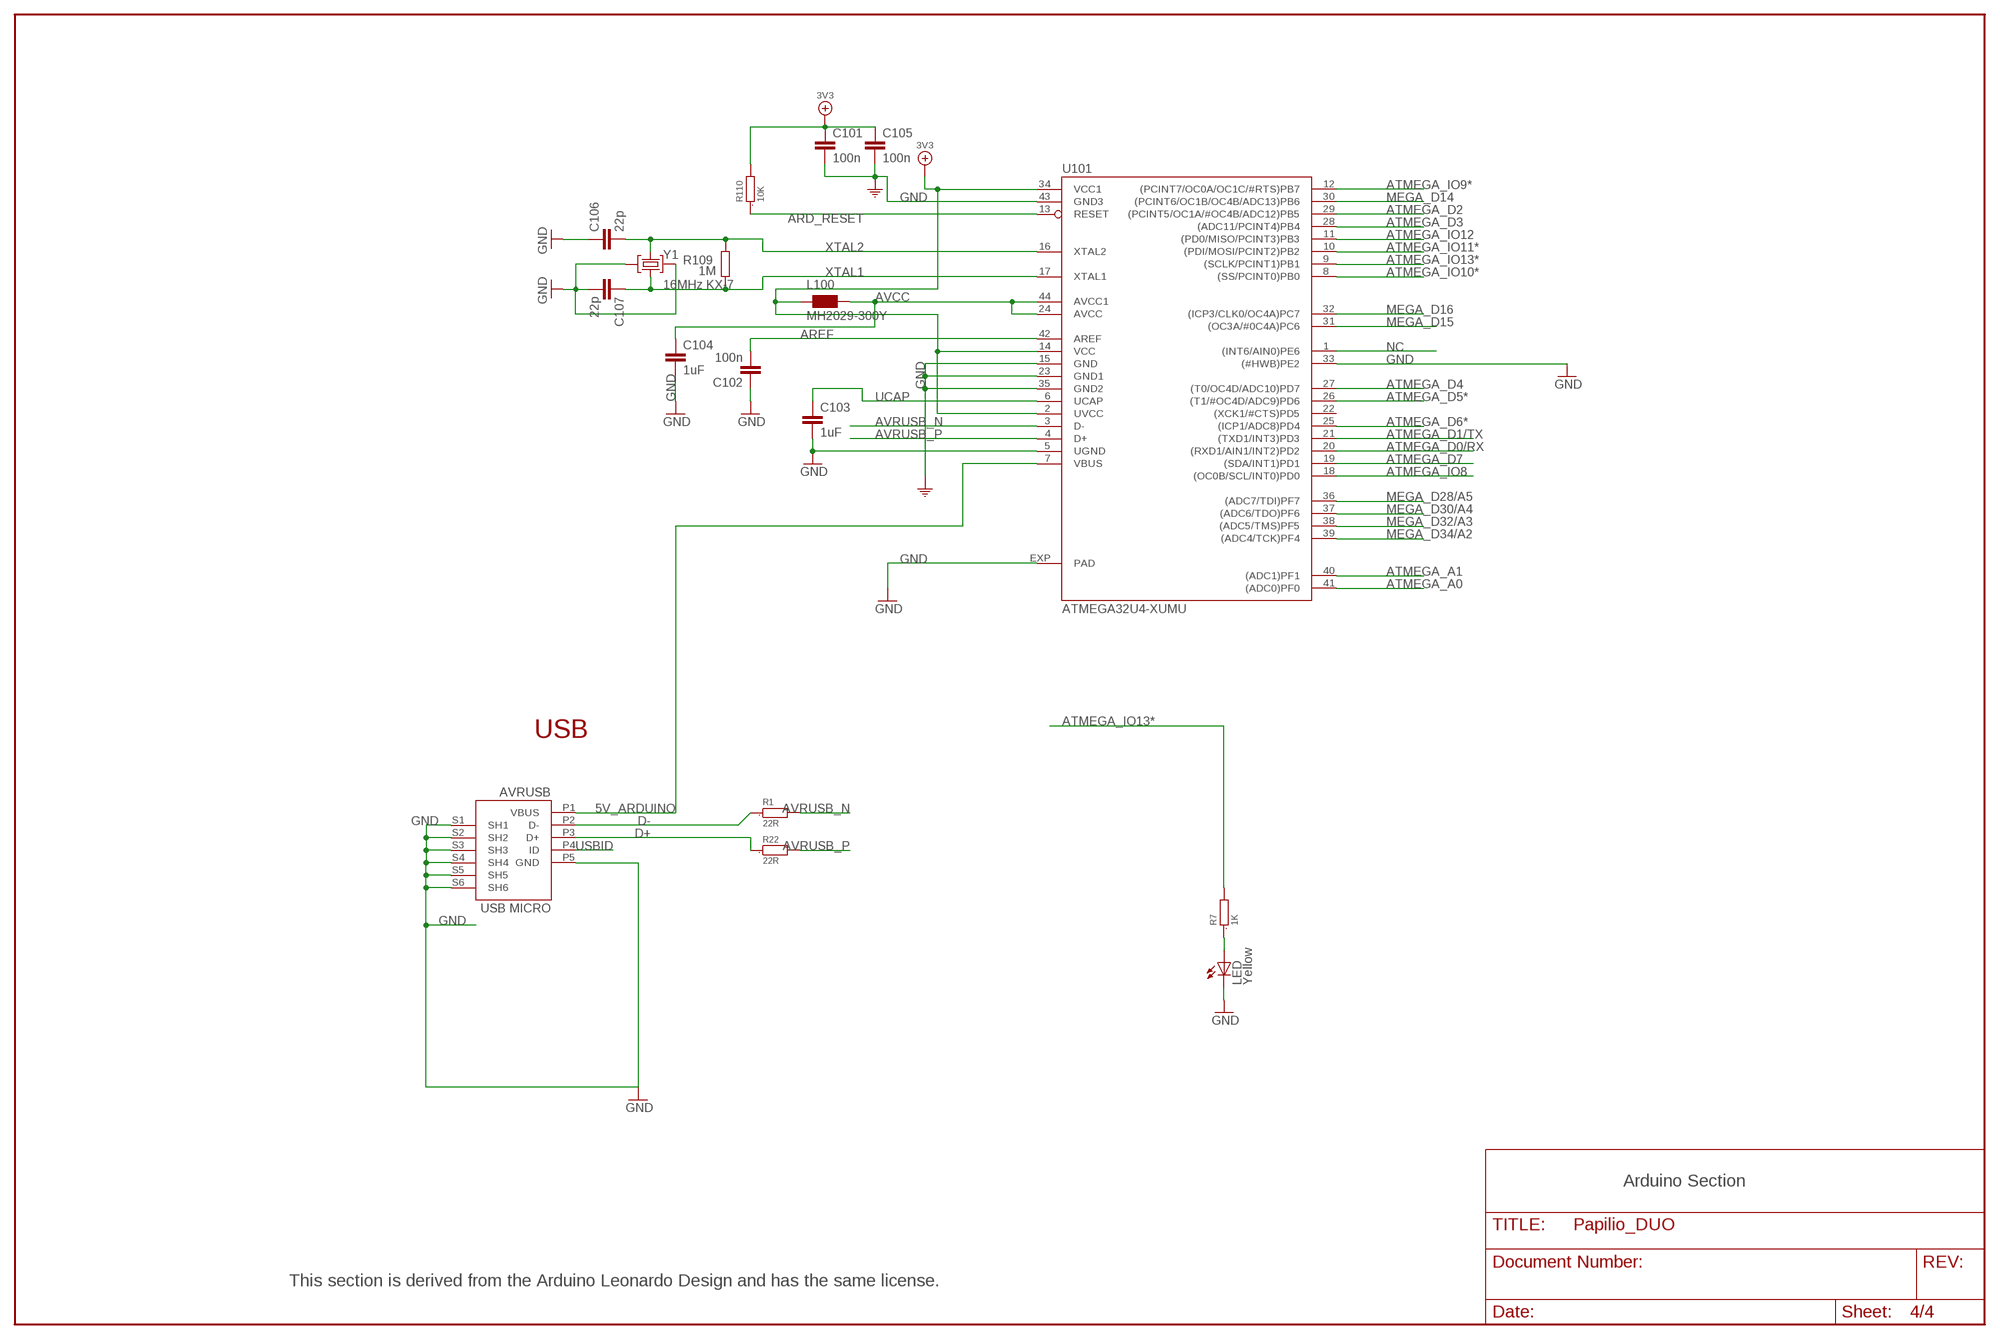
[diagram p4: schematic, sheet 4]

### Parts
AVRUSB  USB MICRO  MYCON2_USB-MINI-B  [CON2_USB_MICRO_B_AT]
C101  100n  C-EUC0603K  [C0603K]
C102  100n  C-EUC0603K  [C0603K]
C103  1uF  C-EUC0603K  [C0603K]
C104  1uF  C-EUC0603K  [C0603K]
C105  100n  C-EUC0603K  [C0603K]
C106  22p  C-EUC0603K  [C0603K]
C107  22p  C-EUC0603K  [C0603K]
L100  MH2029-300Y  WE-CBF_0805  [0805]
LED  Yellow  LEDCHIPLED_0805  [CHIPLED_0805]
R1  22R  R0805  [0805]
R7  1K  R0603  [0603]
R22  22R  R0805  [0805]
R109  1M  R-EU_R0603  [R0603-ROUND]
R110  10K  R0603  [0603]
U101  ATMEGA32U4-XUMU  [QFN44ML7X7]
Y1  16MHz KX-7  CRYSTAL-3.2-2.5  [CRYSTAL-3.2-2.5]

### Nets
3V3: C101.1 C105.1 L100.1 R110.2 U101.2(UVCC) U101.14(VCC) U101.34(VCC1) ; also sheet 1,2,3
5V_ARDUINO: AVRUSB.P1(VBUS) U101.7(VBUS) ; also sheet 2
ARD_RESET: R110.1 U101.13(RESET) ; also sheet 1
AREF [aref]: C102.2 U101.42(AREF) ; also sheet 1
ATMEGA_A0: U101.41((ADC0)PF0) ; also sheet 1
ATMEGA_A1: U101.40((ADC1)PF1) ; also sheet 1
ATMEGA_D0/RX: U101.20((RXD1/AIN1/INT2)PD2) ; also sheet 1
ATMEGA_D1/TX: U101.21((TXD1/INT3)PD3) ; also sheet 1
ATMEGA_D2: U101.29((PCINT5/OC1A/#OC4B/ADC12)PB5) ; also sheet 1
ATMEGA_D3: U101.28((ADC11/PCINT4)PB4) ; also sheet 1
ATMEGA_D4: U101.27((T0/OC4D/ADC10)PD7) ; also sheet 1
ATMEGA_D5*: U101.26((T1/#OC4D/ADC9)PD6) ; also sheet 1
ATMEGA_D6*: U101.25((ICP1/ADC8)PD4) ; also sheet 1
ATMEGA_D7: U101.19((SDA/INT1)PD1) ; also sheet 1
ATMEGA_IO8: U101.18((OC0B/SCL/INT0)PD0) ; also sheet 1
ATMEGA_IO9*: U101.12((PCINT7/OC0A/OC1C/#RTS)PB7) ; also sheet 1
ATMEGA_IO10*: U101.8((SS/PCINT0)PB0) ; also sheet 1
ATMEGA_IO11*: U101.10((PDI/MOSI/PCINT2)PB2) ; also sheet 1
ATMEGA_IO12: U101.11((PD0/MISO/PCINT3)PB3) ; also sheet 1
ATMEGA_IO13*: R7.2 U101.9((SCLK/PCINT1)PB1) ; also sheet 1
AVCC: C104.1 L100.2 U101.24(AVCC) U101.44(AVCC1)
AVRUSB_N: R1.2 U101.3(D-)
AVRUSB_P: R22.2 U101.4(D+)
D+: AVRUSB.P3(D+) R22.1
D-: AVRUSB.P2(D-) R1.1
GND: AVRUSB.P5(GND) AVRUSB.S1(SH1) AVRUSB.S2(SH2) AVRUSB.S3(SH3) AVRUSB.S4(SH4) AVRUSB.S5(SH5) AVRUSB.S6(SH6) C101.2 C102.1 C103.2 C104.2 C105.2 C106.1 C107.2 LED.C U101.5(UGND) U101.15(GND) U101.23(GND1) U101.33((#HWB)PE2) U101.35(GND2) U101.43(GND3) U101.EXP(PAD) Y1.2(GND) Y1.4(GND) ; supply symbol labelled COM ; also sheet 1,2,3
MEGA_D14: U101.30((PCINT6/OC1B/OC4B/ADC13)PB6) ; also sheet 1
MEGA_D15: U101.31((OC3A/#0C4A)PC6) ; also sheet 1
MEGA_D16: U101.32((ICP3/CLK0/OC4A)PC7) ; also sheet 1
MEGA_D28/A5: U101.36((ADC7/TDI)PF7) ; also sheet 1
MEGA_D30/A4: U101.37((ADC6/TDO)PF6) ; also sheet 1
MEGA_D32/A3: U101.38((ADC5/TMS)PF5) ; also sheet 1
MEGA_D34/A2: U101.39((ADC4/TCK)PF4) ; also sheet 1
N$2: LED.A R7.1
NC: U101.1((INT6/AIN0)PE6)
UCAP: C103.1 U101.6(UCAP)
USBID: AVRUSB.P4(ID)
XTAL1: C107.1 R109.1 U101.17(XTAL1) Y1.1(C1)
XTAL2: C106.2 R109.2 U101.16(XTAL2) Y1.3(C2)
Unconnected: U101.22((XCK1/#CTS)PD5)

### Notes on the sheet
- USB
- Arduino Section
- This section is derived from the Arduino Leonardo Design and has the same license.

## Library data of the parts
AVRUSB = SmartPrj:MYCON2_USB-MINI-B; PARTNO: 10118193-0001LF
C1 C2 = Bogdan_Commons:C: CAPACITOR, European symbol; PARTNO: GRM21BR60J226ME39L
C3 = Bogdan_Commons:C: CAPACITOR, European symbol; PARTNO: C0805C106K9PACTU
C4-C7 C10-C13 C21-C26 C32 C33 C35 C36 = GadgetFactory:C: CAPACITOR, European symbol; PARTNO: GRM188F51E104ZA01D
C8 C9 = dp_devices:CAP; PARTNO: CL10C270JB8NNNC
C14 C28 = dp_devices:CAP_POL; PARTNO: T491A475M010AT
C15-C18 C20 C27 C29-C31 C34 = dp_devices:CAP; PARTNO: GRM188F51E104ZA01D
C19 = dp_devices:CAP_POL; PARTNO: T491A335K016AT7280
C101 C102 C105 = SmartPrj:C-EU: CAPACITOR, European symbol; PARTNO: GRM188F51E104ZA01D
C103 C104 = SmartPrj:C-EU: CAPACITOR, European symbol; PARTNO: C1608X5R1A105K080AC
C106 C107 = SmartPrj:C-EU: CAPACITOR, European symbol; PARTNO: C1608C0G1H220J080AA
FLASH = GadgetFactory:FLASH-SPI-25XX: SPI Flash; PARTNO: MX25L6445EM2I-10G
FPGAUSB = dp_devices:CONN_USB: USB connector; PARTNO: USB-M26FTR
IC1 = DP-EagleLibrary:FT2232H: DUAL HIGH SPEED USB TO MULTIPURPOSE UART/FIFO IC; PARTNO: FT2232HL-REEL
L1 L2 = Bogdan_Commons:L: INDUCTOR, European symbol; PARTNO: VLS3015T-3R3M1R2
L3 L4 = dp_devices:FERRITE_BEAD; PARTNO: MMZ1608R600A
L100 = wuerth-elektronik:WE-CBF: SMD EMI Suppression Ferrite Beads; PARTNO: MH2029-300YCT-ND
LED = led:LED: LED; PARTNO: LTST-C170KGKT
OSC = MondoCPLDCore-XC95_Rev1.5:OSC1; PARTNO: ASV-32.000MHZ-E-T
PWR = led:LED: LED; PARTNO: LTST-C171EKT
PWRIN = jumper:JP1E: JUMPER; PARTNO: 68000-102HLF
PWRSEL = jumper:JP2E: JUMPER; PARTNO: 68000-103HLF
R1 R22 = GadgetFactory_6.0:R: RESISTOR, European symbol; PARTNO: RMCF0805JT22R0
R2 = Bogdan_Commons:R-SMALL; PARTNO: CRCW06036K80FKEA
R3-R5 = Bogdan_Commons:R-SMALL; PARTNO: CRCW06031K50FKEA
R6 = GadgetFactory:R: RESISTOR, European symbol; PARTNO: RMCF0603JT1K80
R7 = GadgetFactory_6.0:R: RESISTOR, European symbol; PARTNO: RMCF0603JT1K00
R8-R21 = GadgetFactory:R: RESISTOR, European symbol; PARTNO: RMCF0603JT390R
R23 R24 R26 R28 = dp_devices:RESISTOR; PARTNO: RMCF0603JT10K0
R25 = dp_devices:RESISTOR; PARTNO: RMCF0603JT2K20
R27 = dp_devices:RESISTOR; PARTNO: RMCF0603FT12K0
R29 R30 = dp_devices:RESISTOR; PARTNO: RMCF0603JT470R
R31 = GadgetFactory:R: RESISTOR, European symbol; PARTNO: RMCF0805JT47K0
R32 = GadgetFactory:R: RESISTOR, European symbol; PARTNO: RMCF0603JT4K70
R109 = SmartPrj:R-EU_: RESISTOR, European symbol; PARTNO: RMCF0603JT1M00
R110 = GadgetFactory_6.0:R: RESISTOR, European symbol; PARTNO: RMCF0603JT10K0
RX TX = dp_devices:LED; PARTNO: LTST-C170KGKT
S1 = xilinx_devices:6SLX9TQG144: Xilinx FPGA: 6SLX9TQG144; PARTNO: XC6SLX9-2TQG144C
SRAM = GadgetFactory:ISSI_SRAM_8BIT; PARTNO: IS61WV20488BLL-10TLI
SW1 = OPL Eagle Library:SWITCH-2CH-6P*: MS-22D18 G2 ROHS; PARTNO: EG1271
SW2 = adafruit:EVQQ2: SMT 6mm switch, EVQQ2 series http://www.ladyada.net/library/eagle; PARTNO: PTS525SM10SMTR LFS
U1 = GadgetFactory_tmp:ARDUINO_MEGA_SHIELD; BOM: EXCLUDE
U2 = Bogdan_Commons:LTC3419: Dual Monolithic 600mA Synchronous Step-Down Regulator; PARTNO: LTC3419EMS#PBF
U3 = Bogdan_Commons:DIGITAL-EEPROM-MICROWIRE-6P; PARTNO: 93C46BT-I/OT
U101 = SmartPrj:ATMEGA32U4-XU; PARTNO: ATMEGA32U4RC-MUR
U$1 = GadgetFactory:JTAG_XILINX; BOM: EXCLUDE
WING_POWER1-WING_POWER6 = Papilio:POWER_ONLY; PARTNO: PPTC041LFBN-RC
X1 = dp_devices:CRYSTAL_2; PARTNO: ABM7-12.000MHZ-D2Y-T
Y1 = SmartPrj:CRYSTAL-3.2-2.5; PARTNO: ABM8G-16.000MHZ-B4Y-T

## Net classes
0 default: width 0.178 mm, drill 0.381 mm, clearance 0.178 mm
1 Power: width 0.254 mm, drill 0.381 mm, clearance 0.178 mm
2 gnd: width 0.254 mm, drill 0.61 mm, clearance 0.254 mm
3 usbvcc: width 0.254 mm, drill 0.61 mm, clearance 0.254 mm
4 aref: width 0.254 mm, drill 0.61 mm, clearance 0.254 mm

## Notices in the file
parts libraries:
bom: Copyright (C) 2010, Bob Starr
SparkFun-Aesthetics: Licensing: CC v3.0 Share-Alike You are welcome to use this library for commercial purposes.
